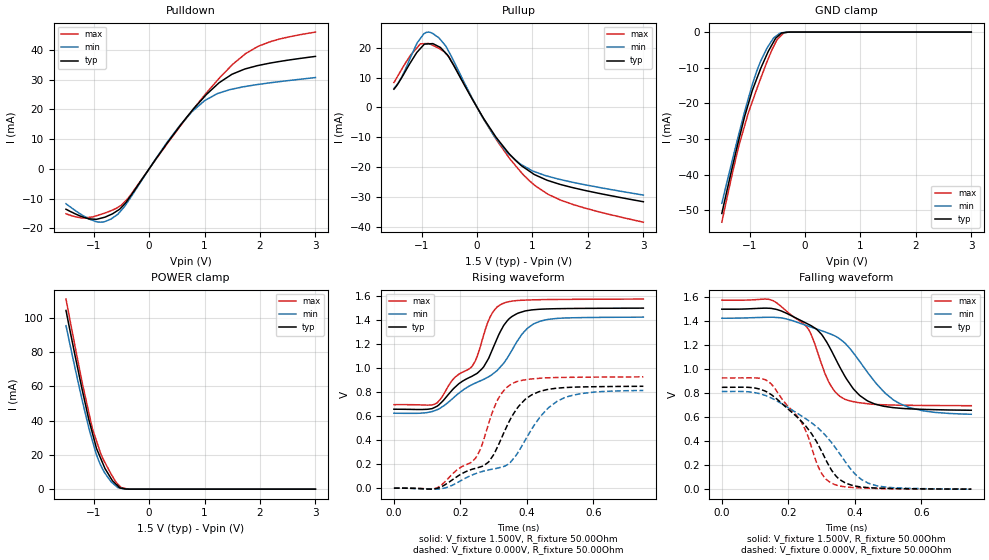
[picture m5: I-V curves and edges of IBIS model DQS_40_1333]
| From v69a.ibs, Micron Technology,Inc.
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| MODEL DQS_40_1333 (40 Ohm Data Strobe I/O with no ODT, 1333Mbps)
[Model]   DQS_40_1333
Model_type   I/O
Vinl = 600.000mV
Vinh = 900.000mV
Vmeas = 750.000mV
Vref = 750.000mV
Cref = 0.0pF
Rref = 25.000Ohm
|   typ   min   max
C_comp   1.25pF   1.10pF   1.39pF
[Model Spec]
| Input threshold voltage corners
Vinl   0.6000V   0.5625V   0.6375V
Vinh   0.9000V   0.8625V   0.9375V
| Measurement voltage corners
Vmeas   0.7500V   0.7125V   0.7875V
| Timing spec test load voltage corners
Vref   0.7500V   0.7125V   0.7875V
|[Receiver Thresholds]
|Vth   =  0.750V
|Vth_min  =  0.735V
|Vth_max  =  0.765V
|Vinh_ac  =  0.150V
|Vinh_dc  =  0.100V
|Vinl_ac  = -0.150V
|Vinl_dc  = -0.100V
|Tslew_ac =  5.000ns |Not specified, so set to high value
|Threshold_sensitivity = 0.50
|Reference_supply Pullup_ref
[Receiver Thresholds]
Vcross_low   = 0.600V
Vcross_high  = 0.900V
Vdiff_ac   = 300mV
Vdiff_dc   = 200mV
Tdiffslew_ac = 10.000ns |Not specified, so set to high value
[Voltage Range]   1.5000V   1.4250V   1.5750V
[Pullup Reference]   1.5000V   1.4250V   1.5750V
| Junction Temperature (Ambient temp is 35C typ, 95C min, 0C max)
[Temperature Range]   50.0   110.0   0.0
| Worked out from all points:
|   slope of the pulldown table from 0 to 0.225 V, typ, clamps not added: 37.3 ohm
|   slope of the pullup table from 0 to 0.225 V, typ, clamps not added: 33.3 ohm
|   GND clamp passes 1 mA (typ) near -0.48 V on its own axis
|   POWER clamp passes 1 mA (typ) near -0.54 V on its own axis
|   falling waveform, V_fixture 1.500V, R_fixture 50.00Ohm: 20-80 % time 113ps typ, 150ps min, 90.4ps max; typ from 1.5 V to 0.657 V
|   rising waveform, V_fixture 1.500V, R_fixture 50.00Ohm: 20-80 % time 147ps typ, 188ps min, 116ps max; typ from 0.657 V to 1.5 V
|   rising waveform, V_fixture 0.000V, R_fixture 50.00Ohm: 20-80 % time 123ps typ, 153ps min, 104ps max; typ from 0 V to 0.848 V
|   falling waveform, V_fixture 0.000V, R_fixture 50.00Ohm: 20-80 % time 133ps typ, 173ps min, 107ps max; typ from 0.848 V to 0 V
[Pulldown]
|   Voltage   I(typ)   I(min)   I(max)
-1.5V     -13.6mA    -11.75mA   -15.12mA
-1.195V   -16.21mA   -15.72mA   -16.58mA
-960mV    -16.98mA   -17.75mA   -15.83mA
-690mV    -15.38mA   -16.91mA   -14.11mA
-530mV    -13.56mA   -14.54mA   -12.57mA
-380mV    -10.33mA   -10.94mA   -9.938mA
540mV     14.03mA    14.24mA    13.81mA
1V        24.29mA    22.9mA     24.74mA
1.265V    28.96mA    25.48mA    30.46mA
1.495V    31.78mA    26.77mA    34.87mA
1.97V     34.74mA    28.36mA    41.2mA
3V        37.78mA    30.67mA    45.95mA
[GND Clamp]
|   Voltage   I(typ)   I(min)   I(max)
-1.5V     -50.86mA   -48.03mA   -53.31mA
-1.32V    -38.49mA   -36.47mA   -40.31mA
-1.195V   -30.28mA   -28.67mA   -32mA
-1.085V   -23.47mA   -22.1mA    -26.06mA
-950mV    -16.36mA   -14.72mA   -19.5mA
-875mV    -13.3mA    -11.18mA   -16.21mA
-805mV    -10.44mA   -8.35mA    -13.23mA
-690mV    -6.381mA   -4.61mA    -8.515mA
-565mV    -2.71mA    -1.629mA   -4.002mA
-505mV    -1.389mA   -935.1uA   -2.13mA
-380mV    -171.4uA   -110.2uA   -180.2uA
3V        0A         0A         0A
[Pullup]
|   Voltage   I(typ)   I(min)   I(max)
-1.5V     6.153mA    6.385mA    8.388mA
-1.365V   9.878mA    9.978mA    12.67mA
-1.025V   19.77mA    23.13mA    21.32mA
-835mV    21.43mA    25.16mA    21.21mA
-660mV    20.15mA    22.79mA    19.54mA
-505mV    16.8mA     18.6mA     16.93mA
80mV      -2.482mA   -2.723mA   -2.581mA
310mV     -9.086mA   -9.637mA   -9.633mA
770mV     -19.05mA   -18.9mA    -21.22mA
1.055V    -22.71mA   -21.69mA   -26.38mA
1.51V     -25.9mA    -24.24mA   -31.14mA
3V        -31.67mA   -29.44mA   -38.55mA
[POWER Clamp]
|   Voltage   I(typ)   I(min)   I(max)
-1.5V     104.2mA    95.33mA    110.8mA
-1.195V   56.08mA    50.05mA    60.2mA
-1.09V    40.77mA    35.95mA    44.95mA
-1.025V   32.84mA    28.43mA    35.51mA
-950mV    23.76mA    20.16mA    28.1mA
-870mV    17.62mA    13.67mA    20.38mA
-795mV    11.95mA    9.2mA      15.38mA
-690mV    6.402mA    4.437mA    8.988mA
-595mV    2.805mA    1.754mA    3.913mA
-505mV    588.2uA    491.1uA    931.8uA
-300mV    1.53uA     2.94uA     1.674uA
3V        0A         0A         0A
[Ramp]
R_load = 50.00Ohm
|   typ   min   max
dV/dt_r   508.798mV/122.874ps 487.677mV/153.148ps 555.841mV/104.130ps
dV/dt_f   504.967mV/113.369ps 479.854mV/150.024ps 527.439mV/90.394ps
[Falling Waveform]
V_fixture = 1.500V
V_fixture_min = 1.425V
V_fixture_max = 1.575V
R_fixture = 50.00Ohm
|   Time   V(typ)   V(min)   V(max)
0s        1.499V     1.424V     1.574V
145ps     1.506V     1.432V     1.578V
245ps     1.394V     1.372V     1.38V
270ps     1.359V     1.348V     1.279V
325ps     1.176V     1.294V     874.9mV
370ps     940.3mV    1.217V     748.6mV
435ps     740.5mV    984.6mV    712.8mV
525ps     676.7mV    728.3mV    700mV
605ps     664.6mV    652.3mV    697.3mV
750ps     657.2mV    623.8mV    695.1mV
[Rising Waveform]
V_fixture = 1.500V
V_fixture_min = 1.425V
V_fixture_max = 1.575V
R_fixture = 50.00Ohm
|   Time   V(typ)   V(min)   V(max)
0s        657.2mV    623.8mV    695.1mV
130ps     682.3mV    653mV      710.6mV
185ps     843.5mV    767mV      926.7mV
235ps     932mV      861.9mV    1.014V
270ps     1.011V     905.8mV    1.277V
290ps     1.115V     935.6mV    1.429V
325ps     1.329V     1.024V     1.534V
385ps     1.467V     1.282V     1.564V
440ps     1.49V      1.391V     1.569V
750ps     1.499V     1.424V     1.574V
[Rising Waveform]
V_fixture = 0.000V
V_fixture_min = 0.000V
V_fixture_max = 0.000V
R_fixture = 50.00Ohm
|   Time   V(typ)   V(min)   V(max)
0s        250uV      307.8uV    134.6uV
130ps     -1.608mV   -7.595mV   2.595mV
235ps     157.3mV    109.2mV    219.7mV
260ps     177.2mV    134.3mV    324mV
285ps     218.8mV    151.8mV    539.9mV
320ps     395mV      172.8mV    774.5mV
355ps     598.7mV    231.2mV    870mV
415ps     777.9mV    494.5mV    909.4mV
490ps     832.2mV    722.2mV    921mV
750ps     848.2mV    813.1mV    926.5mV
[Falling Waveform]
V_fixture = 0.000V
V_fixture_min = 0.000V
V_fixture_max = 0.000V
R_fixture = 50.00Ohm
|   Time   V(typ)   V(min)   V(max)
0s        848.2mV    813.1mV    926.5mV
100ps     842.2mV    803.4mV    926.8mV
145ps     793.9mV    763.7mV    885mV
250ps     533.6mV    591.1mV    500.3mV
295ps     342.3mV    494.4mV    156.6mV
335ps     138.8mV    369.7mV    43.81mV
360ps     70.55mV    272.6mV    23.82mV
400ps     26.75mV    127.4mV    12.87mV
445ps     12.4mV     45.75mV    7.306mV
750ps     250uV      307.8uV    134.6uV
